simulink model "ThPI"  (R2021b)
settings: Solver=FixedStepAuto  StartTime=0  StopTime=timeWaypoints(end)-0.2  FixedStep=0.005  RelTol=1e-3
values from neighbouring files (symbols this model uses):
  a = 0.27    [CompareGazeboSimulink.m]    (also in RobotModel.m)
  b = 0.31    [CompareGazeboSimulink.m]    (also in RobotModel.m)
  D = abs(a-b)    [RobotModel.m]
  Dflag = 1    [RobotModel.m]
  distAng = 0    [RobotModel.m]
  distVel = 0    [RobotModel.m]
  fro = 0.02    [CompareGazeboSimulink.m]    (also in RobotModel.m)
  fsl = 0.8    [CompareGazeboSimulink.m]    (also in RobotModel.m)
  fsly = 0.8    [CompareGazeboSimulink.m]    (also in RobotModel.m)
  I = (1/12)*m*((2*t)^2 + 0.12^2) + 1.5    (= 2.384)    [CompareGazeboSimulink.m]    (also in RobotModel.m = 0.866666666667)
  Iflag = 1    [RobotModel.m]
  K = 22    [RobotModel.m]
  ko = 0    [CompareGazeboSimulink.m]    (also in RobotModel.m = 0.25)
  kt = 0.58    [CompareGazeboSimulink.m]    (also in RobotModel.m)
  kx = 0.5    [RobotModel.m]
  ky = 0.5    [RobotModel.m]
  lx = 0.15    [RobotModel.m]
  ly = 0.15    [RobotModel.m]
  m = 51    [CompareGazeboSimulink.m]    (also in RobotModel.m = 50)
  mdy = 10    [CompareGazeboSimulink.m]    (also in RobotModel.m)
  mst = 10    [CompareGazeboSimulink.m]    (also in RobotModel.m)
  N = 0    [RobotModel.m]
  r = 0.19    [CompareGazeboSimulink.m]    (also in RobotModel.m)
  T_vel_variance = 0.0005    [RobotModel.m]
  Td = 0.0125    [RobotModel.m]
  Th0 = 0    [CompareGazeboSimulink.m]    (also in RobotModel.m = 0.9714)
  Th_vel0 = 0    [CompareGazeboSimulink.m]    (also in RobotModel.m)
  Ti = 0.1    [RobotModel.m]
  timeWaypoints = [0, 3, 7.5, 10.5, 13.5, 18, 20.5]    [RobotModel.m]
  Ts = 0.01    [CompareGazeboSimulink.m]    (also in RobotModel.m = 0.05)
  waypoints = [0 5; 4 9; 8 1; 12 5; 8 9; 4 1; 0 5]    [CubicSpline.m]    (also in RobotModel.m = [0 2.5; 2 4.5; 4 0.5; 6 2.5; 4 4.5; 2 0.5; 0 2.5])
  X0 = 0    [CompareGazeboSimulink.m]    (also in RobotModel.m)
  x_vel0 = 0    [CompareGazeboSimulink.m]    (also in RobotModel.m)
  x_vel_variance = 0.0005    [RobotModel.m]
  Y0 = 0    [CompareGazeboSimulink.m]    (also in RobotModel.m = 2.5)

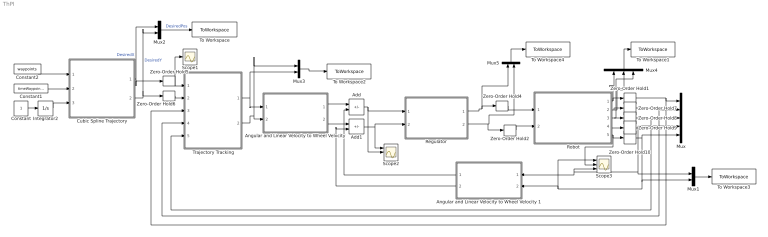
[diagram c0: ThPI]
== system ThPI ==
  Add : Sum  Inputs=+-
  Add1 : Sum  Inputs=+-
  Angular and Linear Velocity to Wheel Velocity : Subsystem
  Angular and Linear Velocity to Wheel Velocity 1 : Subsystem
  Constant : Constant
  Constant1 : Constant  Value=timeWaypoints
  Constant2 : Constant  Value=waypoints
  Cubic Spline Trajectory : MATLAB Function  TreatAsAtomicUnit=on
  Integrator2 : Integrator
  Mux : Mux  Inputs=5
  Mux{1..3,5} (4 alike) : Mux  Inputs=2
  Mux4 : Mux  Inputs=3
  Regulator : Subsystem
  Robot : Subsystem
  Scope1 : Scope
  Scope2 : Scope  NumInputPorts=3
  Scope3 : Scope  NumInputPorts=3
  To Workspace : ToWorkspace  VariableName=desiredPos  SaveFormat=Timeseries  SampleTime=-1
  To Workspace1 : ToWorkspace  VariableName=ActualPos  SaveFormat=Timeseries  SampleTime=-1
  To Workspace2 : ToWorkspace  VariableName=DesiredVel  SaveFormat=Timeseries  SampleTime=-1
  To Workspace3 : ToWorkspace  VariableName=ActualVel  SaveFormat=Timeseries  SampleTime=-1
  To Workspace4 : ToWorkspace  VariableName=Forces  SaveFormat=Timeseries  SampleTime=-1
  Trajectory Tracking : Subsystem
  Zero-Order Hold{1..2,4..10} (9 alike) : ZeroOrderHold  SampleTime=Ts
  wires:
  Angular and Linear Velocity to Wheel Velocity 1/1(wl) -> Add/2
  Angular and Linear Velocity to Wheel Velocity 1/2("wr ") -> Add1/2
  Constant2/1 -> Cubic Spline Trajectory/1(waypoints)
  Constant/1 -> Integrator2/1
  Constant1/1 -> Cubic Spline Trajectory/2(time)
  Integrator2/1 -> Cubic Spline Trajectory/3(actualTime)
  Cubic Spline Trajectory/1(X) -> Mux2/1, Zero-Order Hold5/1  "DesiredX"
  Cubic Spline Trajectory/2(Y) -> Zero-Order Hold6/1, Mux2/2  "DesiredY"
  Add/1 -> Scope2/2, Regulator/1(wl)
  Add1/1 -> Scope2/1, Regulator/2(wr)
  Regulator/2(Right force action) -> Mux5/2, Zero-Order Hold2/1
  Regulator/1(Left Force action) -> Mux5/1, Zero-Order Hold4/1
  Angular and Linear Velocity to Wheel Velocity/1(wl) -> Add/1
  Angular and Linear Velocity to Wheel Velocity/2("wr ") -> Add1/1
  Zero-Order Hold4/1 -> Robot/1(Left Force)
  Zero-Order Hold2/1 -> Robot/2(Right Force)
  Mux2/1 -> To Workspace/1  "DesiredPos"
  Zero-Order Hold5/1 -> Scope1/1, Trajectory Tracking/1(Xd)
  Zero-Order Hold6/1 -> Trajectory Tracking/2(Yd)
  Mux4/1 -> To Workspace1/1
  Robot/1(X) -> Mux4/1, Zero-Order Hold1/1
  Robot/2(Y) -> Mux4/2, Zero-Order Hold7/1
  Robot/5(v) -> Scope3/2, Zero-Order Hold10/1
  Zero-Order Hold8/1 -> Trajectory Tracking/5(Theta), Mux/3
  Zero-Order Hold10/1 -> Scope3/1, Angular and Linear Velocity to Wheel Velocity 1/2(Linear Velocity), Mux1/2, Mux/5
  Zero-Order Hold9/1 -> Scope3/3, Angular and Linear Velocity to Wheel Velocity 1/1(Angular Velocity), Mux1/1, Mux/4
  Zero-Order Hold1/1 -> Trajectory Tracking/3(X), Mux/1
  Zero-Order Hold7/1 -> Trajectory Tracking/4(Y), Mux/2
  Robot/3(Theta) -> Mux4/3, Zero-Order Hold8/1
  Robot/4(Theta') -> Zero-Order Hold9/1
  Mux5/1 -> To Workspace4/1
  Mux1/1 -> To Workspace3/1
  Mux3/1 -> To Workspace2/1
  Trajectory Tracking/1(" Linear Velocity") -> Mux3/2, Angular and Linear Velocity to Wheel Velocity/1(Linear Velocity)
  Trajectory Tracking/2(Angular Velocity) -> Mux3/1, Angular and Linear Velocity to Wheel Velocity/2(Angular Velocity)

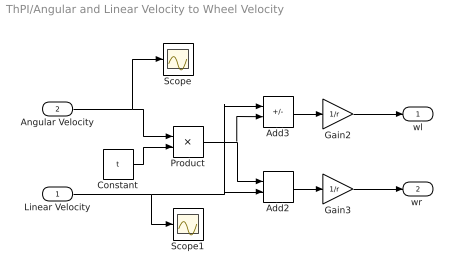
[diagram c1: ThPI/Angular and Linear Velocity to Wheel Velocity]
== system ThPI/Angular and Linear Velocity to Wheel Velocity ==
  Linear Velocity : Inport
  Angular Velocity : Inport  Port=2
  Add2 : Sum
  Add3 : Sum  Inputs=+-
  Constant : Constant  Value=t
  Gain2 : Gain  Gain=1/r
  Gain3 : Gain  Gain=1/r
  Product : Product
  Scope : Scope
  Scope1 : Scope
  wl : Outport
  "wr " : Outport  Port=2
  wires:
  Gain2/1 -> wl/1
  Linear Velocity/1 -> Scope1/1, Add2/2, Add3/1
  Gain3/1 -> "wr "/1
  Product/1 -> Add3/2, Add2/1
  Constant/1 -> Product/2
  Add3/1 -> Gain2/1
  Add2/1 -> Gain3/1
  Angular Velocity/1 -> Scope/1, Product/1

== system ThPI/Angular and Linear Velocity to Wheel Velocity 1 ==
  Angular Velocity : Inport
  Linear Velocity : Inport  Port=2
  Add2 : Sum
  Add3 : Sum  Inputs=+-
  Constant : Constant  Value=t
  Gain2 : Gain  Gain=1/r
  Gain3 : Gain  Gain=1/r
  Product : Product
  wl : Outport
  "wr " : Outport  Port=2
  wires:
  Angular Velocity/1 -> Product/1
  Add2/1 -> Gain3/1
  Add3/1 -> Gain2/1
  Constant/1 -> Product/2
  Product/1 -> Add2/1, Add3/2
  Gain3/1 -> "wr "/1
  Linear Velocity/1 -> Add3/1, Add2/2
  Gain2/1 -> wl/1

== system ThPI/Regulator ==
  wl : Inport
  wr : Inport  Port=2
  PSDN : Subsystem
  PSDN1 : Subsystem
  Left Force action : Outport
  Right force action : Outport  Port=2
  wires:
  wl/1 -> PSDN/1(wl)
  PSDN/1(Left Force action) -> Left Force action/1
  wr/1 -> PSDN1/1(wr)
  PSDN1/1(Right force action) -> Right force action/1

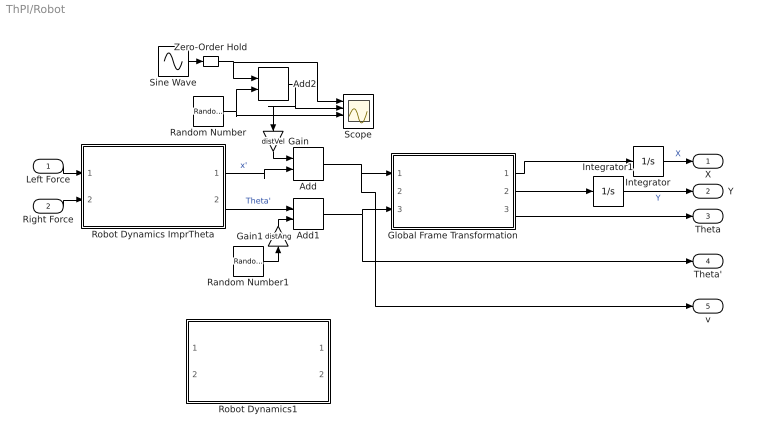
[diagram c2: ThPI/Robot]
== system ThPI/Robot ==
  Left Force : Inport
  Right Force : Inport  Port=2
  Add : Sum
  Add1 : Sum
  Add2 : Sum
  Gain : Gain  Gain=distVel
  Gain1 : Gain  Gain=distAng
  Global Frame Transformation : Subsystem
  Integrator : Integrator  InitialCondition=X0
  Integrator1 : Integrator  InitialCondition=Y0
  Random Number : RandomNumber  Variance=x_vel_variance  SampleTime=0.5
  Random Number1 : RandomNumber  Variance=T_vel_variance  SampleTime=0.1
  Robot Dynamics ImprTheta : Subsystem
  Robot Dynamics1 : Subsystem  Commented=on
  Scope : Scope  NumInputPorts=4
  Sine Wave : Sin  Amplitude=0.1  Frequency=0.2  SampleTime=0
  Zero-Order Hold : ZeroOrderHold  SampleTime=0.25
  X : Outport
  Y : Outport  Port=2
  Theta : Outport  Port=3
  Theta' : Outport  Port=4
  v : Outport  Port=5
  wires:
  Random Number/1 -> Add2/2, Scope/3
  Add2/1 -> Gain/1, Scope/2
  Gain/1 -> Add/1
  Sine Wave/1 -> Zero-Order Hold/1
  Add/1 -> v/1, Global Frame Transformation/1(x')
  Add1/1 -> Theta'/1, Global Frame Transformation/3(Theta')
  Random Number1/1 -> Gain1/1
  Left Force/1 -> Robot Dynamics ImprTheta/1(Left Force)
  Gain1/1 -> Add1/2
  Integrator1/1 -> Y/1  "Y"
  Zero-Order Hold/1 -> Scope/1, Add2/1
  Robot Dynamics ImprTheta/1(x') -> Add/2  "x'"
  Global Frame Transformation/2(Y') -> Integrator1/1
  Integrator/1 -> X/1  "X"
  Right Force/1 -> Robot Dynamics ImprTheta/2(Right Force)
  Global Frame Transformation/1(X') -> Integrator/1
  Global Frame Transformation/3(Theta) -> Theta/1
  Robot Dynamics ImprTheta/2(Theta') -> Add1/1  "Theta'"

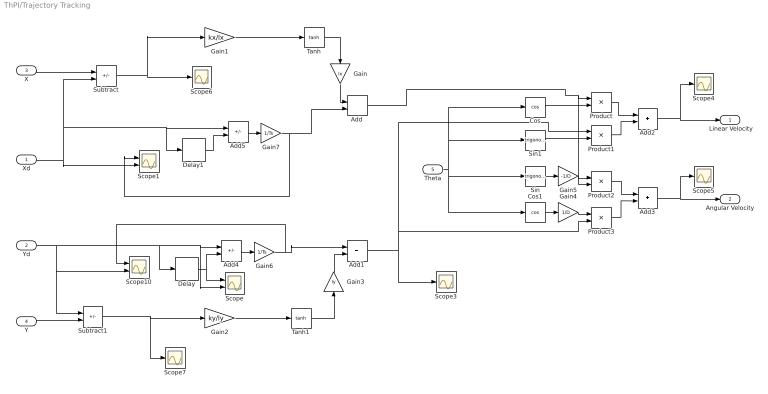
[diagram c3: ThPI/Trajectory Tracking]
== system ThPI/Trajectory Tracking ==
  Xd : Inport
  Yd : Inport  Port=2
  X : Inport  Port=3
  Y : Inport  Port=4
  Theta : Inport  Port=5
  Add{,1..3} (4 alike) : Sum
  Add4 : Sum  Inputs=+-
  Add5 : Sum  Inputs=+-
  Cos : Trigonometry  Operator=cos
  Cos1 : Trigonometry  Operator=cos
  Delay : Delay  DelayLength=1  InitialCondition=Y0
  Delay1 : Delay  DelayLength=1  InitialCondition=X0
  Gain : Gain  Gain=lx
  Gain1 : Gain  Gain=kx/lx
  Gain2 : Gain  Gain=ky/ly
  Gain3 : Gain  Gain=ly
  Gain4 : Gain  Gain=1/D
  Gain5 : Gain  Gain=-1/D
  Gain6 : Gain  Gain=1/Ts
  Gain7 : Gain  Gain=1/Ts
  Product{,1..3} (4 alike) : Product
  Scope : Scope  NumInputPorts=2
  Scope1 : Scope  NumInputPorts=2
  Scope10 : Scope  NumInputPorts=2
  Scope{3..7} (5 alike) : Scope
  Sin : Trigonometry
  Sin1 : Trigonometry
  Subtract : Sum  Inputs=-+
  Subtract1 : Sum  Inputs=+-
  Tanh : Trigonometry  Operator=tanh
  Tanh1 : Trigonometry  Operator=tanh
  " Linear Velocity" : Outport
  Angular Velocity : Outport  Port=2
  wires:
  Subtract/1 -> Gain1/1, Scope6/1
  Subtract1/1 -> Scope7/1, Gain2/1
  Add4/1 -> Gain6/1
  Tanh/1 -> Gain/1
  Gain1/1 -> Tanh/1
  Gain2/1 -> Tanh1/1
  Tanh1/1 -> Gain3/1
  Cos1/1 -> Gain4/1
  Sin/1 -> Gain5/1
  Theta/1 -> Cos/1, Sin1/1, Cos1/1, Sin/1
  Cos/1 -> Product/2
  Add/1 -> Product2/2, Product/1
  Sin1/1 -> Product1/2
  Gain5/1 -> Product2/1
  Gain4/1 -> Product3/1
  Add1/1 -> Scope3/1, Product3/2, Product1/1
  Product/1 -> Add2/1
  Product1/1 -> Add2/2
  Product2/1 -> Add3/1
  Product3/1 -> Add3/2
  Add2/1 -> Scope4/1, " Linear Velocity"/1
  Add3/1 -> Scope5/1, Angular Velocity/1
  Y/1 -> Subtract1/2
  Yd/1 -> Delay/1, Add4/1, Scope/2, Scope10/2, Subtract1/1
  X/1 -> Subtract/1
  Gain/1 -> Add/1
  Gain3/1 -> Add1/2
  Delay/1 -> Scope/1, Add4/2
  Gain6/1 -> Scope10/1, Add1/1
  Gain7/1 -> Scope1/1, Add/2
  Delay1/1 -> Add5/2
  Xd/1 -> Scope1/2, Delay1/1, Add5/1, Subtract/2
  Add5/1 -> Gain7/1

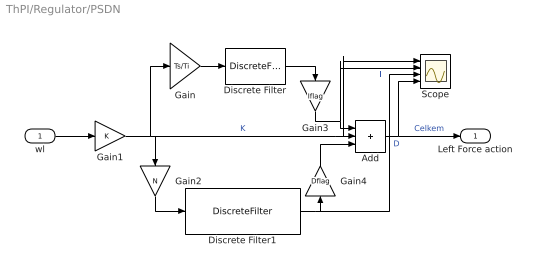
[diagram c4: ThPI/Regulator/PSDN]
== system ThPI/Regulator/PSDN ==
  wl : Inport
  Add : Sum  Inputs=3
  Discrete Filter : DiscreteFilter  Numerator=[0 1]  Denominator=[1 -1]
  Discrete Filter1 : DiscreteFilter  Numerator=[1 -1]  Denominator=[1 -exp(-Ts*N/Td)]
  Gain : Gain  Gain=Ts/Ti
  Gain1 : Gain  Gain=K
  Gain2 : Gain  Gain=N
  Gain3 : Gain  Gain=Iflag
  Gain4 : Gain  Gain=Dflag
  Scope : Scope  NumInputPorts=4
  Left Force action : Outport
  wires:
  Discrete Filter/1 -> Gain3/1
  Discrete Filter1/1 -> Scope/3, Gain4/1  "D"
  wl/1 -> Gain1/1
  Add/1 -> Left Force action/1, Scope/4  "Celkem"
  Gain/1 -> Discrete Filter/1
  Gain1/1 -> Gain2/1, Gain/1, Scope/1, Add/2  "K"
  Gain2/1 -> Discrete Filter1/1
  Gain3/1 -> Scope/2, Add/1  "I"
  Gain4/1 -> Add/3

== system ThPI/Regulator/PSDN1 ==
  wr : Inport
  Add : Sum  Inputs=3
  Discrete Filter : DiscreteFilter  Numerator=[0 1]  Denominator=[1 -1]
  Discrete Filter1 : DiscreteFilter  Numerator=[1 -1]  Denominator=[1 -exp(-Ts*N/Td)]
  Gain : Gain  Gain=Ts/Ti
  Gain1 : Gain  Gain=K
  Gain2 : Gain  Gain=N
  Gain3 : Gain  Gain=Iflag
  Gain4 : Gain  Gain=Dflag
  Right force action : Outport
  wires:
  Gain2/1 -> Discrete Filter1/1
  Gain1/1 -> Add/2, Gain/1, Gain2/1
  Gain/1 -> Discrete Filter/1
  Add/1 -> Right force action/1
  wr/1 -> Gain1/1
  Discrete Filter1/1 -> Gain4/1
  Discrete Filter/1 -> Gain3/1
  Gain3/1 -> Add/1
  Gain4/1 -> Add/3

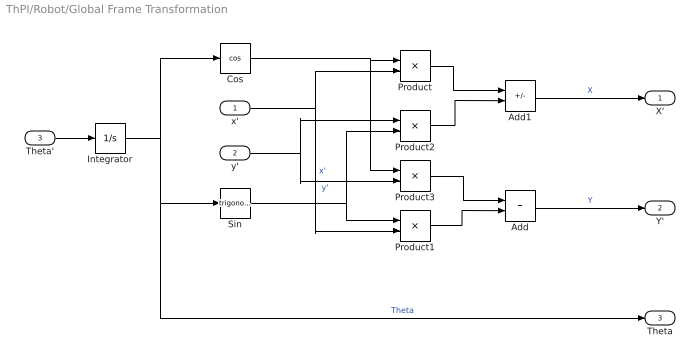
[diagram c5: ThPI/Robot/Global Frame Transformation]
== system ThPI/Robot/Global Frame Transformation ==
  x' : Inport
  y' : Inport  Port=2
  Theta' : Inport  Port=3
  Add : Sum
  Add1 : Sum  Inputs=+-
  Cos : Trigonometry  Operator=cos
  Integrator : Integrator  InitialCondition=Th0
  Product{,1..3} (4 alike) : Product
  Sin : Trigonometry
  X' : Outport
  Y' : Outport  Port=2
  Theta : Outport  Port=3
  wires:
  Add/1 -> Y'/1  "Y"
  Integrator/1 -> Theta/1, Sin/1, Cos/1  "Theta"
  Product1/1 -> Add/2
  x'/1 -> Product/2, Product1/2  "x'"
  Sin/1 -> Product1/1, Product2/2
  Product2/1 -> Add1/2
  Product3/1 -> Add/1
  Product/1 -> Add1/1
  Cos/1 -> Product/1, Product3/1
  y'/1 -> Product3/2, Product2/1  "y'"
  Add1/1 -> X'/1  "X"
  Theta'/1 -> Integrator/1

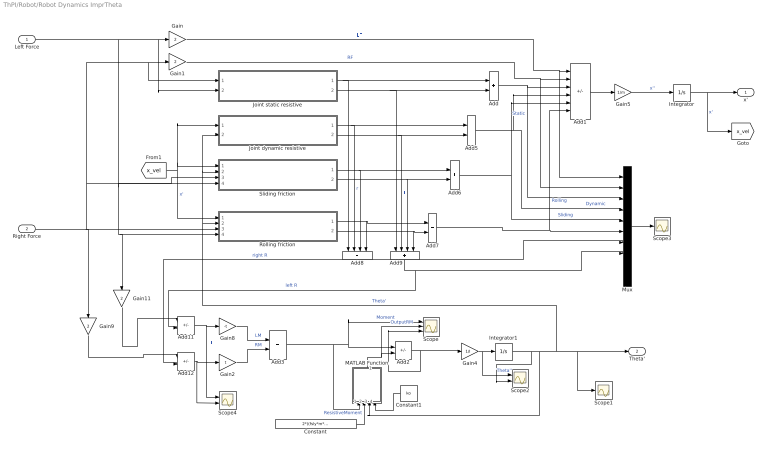
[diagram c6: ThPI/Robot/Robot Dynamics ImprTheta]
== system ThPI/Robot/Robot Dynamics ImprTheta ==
  Left Force : Inport
  Right Force : Inport  Port=2
  Add{,3,5..7} (5 alike) : Sum
  Add1 : Sum  Inputs=++----
  Add11 : Sum  Inputs=+-
  Add12 : Sum  Inputs=+-
  Add2 : Sum  Inputs=+-
  Add8 : Sum  Inputs=++++
  Add9 : Sum  Inputs=++++
  Constant : Constant  Value=2*((fsly*m*9.81)/(a+b))*a*b*kt
  Constant1 : Constant  Value=ko
  Gain{,1,9,11} (4 alike) : Gain  Gain=2
  Gain2 : Gain  Gain=t
  Gain4 : Gain  Gain=1/I
  Gain5 : Gain  Gain=1/m
  Gain8 : Gain  Gain=-t
  Integrator : Integrator  InitialCondition=x_vel0
  Integrator1 : Integrator  InitialCondition=Th_vel0
  Joint dynamic resistive : Subsystem
  Joint static resistive : Subsystem
  MATLAB Function : MATLAB Function  TreatAsAtomicUnit=on
  Mux : Mux  Inputs=10
  Rolling friction : Subsystem
  Scope : Scope  NumInputPorts=3
  Scope1 : Scope
  Scope2 : Scope  NumInputPorts=2
  Scope3 : Scope
  Scope4 : Scope  NumInputPorts=2
  Sliding friction : Subsystem
  x' : Outport
  Theta' : Outport  Port=2
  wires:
  Gain4/1 -> Scope2/1, Integrator1/1  "Theta''"
  Integrator1/1 -> Scope2/2, Sliding friction/2(Theta'), Joint dynamic resistive/2(Theta'), Rolling friction/2(Theta'), Scope1/1, Theta'/1, MATLAB Function/3(Omega)  "Theta'"
  Gain1/1 -> Mux/2, Add1/2  "RF"
  Add1/1 -> Gain5/1
  Gain5/1 -> Integrator/1  "x''"
  Integrator/1 -> x'/1, [x_vel]  "x'"
  [x_vel] -> Joint dynamic resistive/1("Local Long Velocity "), Sliding friction/1(Local longitudal velocity), Rolling friction/1(Local longitudal velocity)  "x'"
  Joint static resistive/2(Static Resistive Force Left) -> Add9/1, Add/2
  Joint dynamic resistive/1(Dynamic Resistive Force Right) -> Add8/2, Add5/1  "r"
  Joint dynamic resistive/2(Dynamic Resistive Force Left) -> Add9/2, Add5/2  "l"
  Sliding friction/1(Friction Right Force) -> Add8/3, Add6/1
  Sliding friction/2(Friction Left Force) -> Add9/3, Add6/2
  Rolling friction/1(Friction Right Force) -> Add8/4, Add7/1
  Rolling friction/2(Friction Left Force) -> Add9/4, Add7/2
  Add/1 -> Add1/3, Mux/3  "Static"
  Add6/1 -> Add1/5, Mux/5  "Sliding"
  Add7/1 -> Mux/6, Add1/6  "Rolling"
  Add5/1 -> Mux/4, Add1/4  "Dynamic"
  Add9/1 -> Add11/2, Mux/8  "left R"
  Add8/1 -> Add12/2, Mux/7  "right R"
  Mux/1 -> Scope3/1
  Add11/1 -> Scope4/1, Gain8/1  "LL"
  Add12/1 -> Scope4/2, Gain2/1
  Gain9/1 -> Add12/1
  Gain11/1 -> Add11/1
  Gain8/1 -> Add3/1  "LM"
  Gain2/1 -> Add3/2  "RM"
  Gain/1 -> Mux/1, Add1/1  "LF"
  Joint static resistive/1(Static Resistive Force Right) -> Add8/1, Add/1
  Add2/1 -> Scope/3, Gain4/1
  Add3/1 -> Scope/1, Add2/1, MATLAB Function/1(Moment)  "Moment"
  MATLAB Function/1(y) -> Scope/2, Add2/2  "OutputRM"
  Constant/1 -> MATLAB Function/2(ResistiveMoment)  "ResistiveMoment"
  Left Force/1 -> Gain11/1, Rolling friction/4(Fl), Sliding friction/4(Fl), Joint static resistive/2("Fl "), Gain/1
  Right Force/1 -> Gain9/1, Rolling friction/3(Fr), Sliding friction/3(Fr), Joint static resistive/1(Fr), Gain1/1
  Constant1/1 -> MATLAB Function/4(ko)

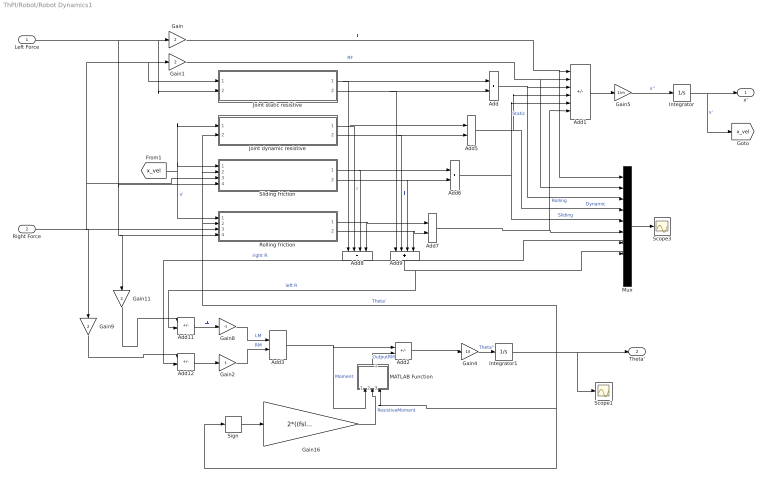
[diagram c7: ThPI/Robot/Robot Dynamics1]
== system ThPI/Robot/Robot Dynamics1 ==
  Left Force : Inport
  Right Force : Inport  Port=2
  Add{,3,5..7} (5 alike) : Sum
  Add1 : Sum  Inputs=++----
  Add11 : Sum  Inputs=+-
  Add12 : Sum  Inputs=+-
  Add2 : Sum  Inputs=+-
  Add8 : Sum  Inputs=++++
  Add9 : Sum  Inputs=++++
  Gain{,1,9,11} (4 alike) : Gain  Gain=2
  Gain16 : Gain  Gain=2*((fsly*m*9.81)/(a+b))*a*b
  Gain2 : Gain  Gain=t
  Gain4 : Gain  Gain=1/I
  Gain5 : Gain  Gain=1/m
  Gain8 : Gain  Gain=-t
  Integrator : Integrator  InitialCondition=x_vel0
  Integrator1 : Integrator  InitialCondition=Th_vel0
  Joint dynamic resistive : Subsystem
  Joint static resistive : Subsystem
  MATLAB Function : MATLAB Function  TreatAsAtomicUnit=on
  Mux : Mux  Inputs=10
  Rolling friction : Subsystem
  Scope1 : Scope
  Scope3 : Scope
  Sign : Signum
  Sliding friction : Subsystem
  x' : Outport
  Theta' : Outport  Port=2
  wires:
  Right Force/1 -> Rolling friction/3(Fr), Sliding friction/3(Fr), Joint static resistive/1(Fr), Gain1/1, Gain9/1
  Gain4/1 -> Integrator1/1  "Theta''"
  Integrator1/1 -> Sliding friction/2(Theta'), Joint dynamic resistive/2(Theta'), Rolling friction/2(Theta'), MATLAB Function/3(Omega), Sign/1, Scope1/1, Theta'/1  "Theta'"
  Left Force/1 -> Rolling friction/4(Fl), Gain11/1, Sliding friction/4(Fl), Joint static resistive/2("Fl "), Gain/1
  Gain1/1 -> Mux/2, Add1/2  "RF"
  Add1/1 -> Gain5/1
  Gain5/1 -> Integrator/1  "x''"
  Integrator/1 -> x'/1, [x_vel]  "x'"
  [x_vel] -> Joint dynamic resistive/1("Local Long Velocity "), Sliding friction/1(Local longitudal velocity), Rolling friction/1(Local longitudal velocity)  "x'"
  Joint static resistive/2(Static Resistive Force Left) -> Add9/1, Add/2
  Joint dynamic resistive/1(Dynamic Resistive Force Right) -> Add8/2, Add5/1  "r"
  Joint dynamic resistive/2(Dynamic Resistive Force Left) -> Add9/2, Add5/2  "l"
  Sliding friction/1(Friction Right Force) -> Add8/3, Add6/1
  Sliding friction/2(Friction Left Force) -> Add9/3, Add6/2
  Rolling friction/1(Friction Right Force) -> Add8/4, Add7/1
  Rolling friction/2(Friction Left Force) -> Add9/4, Add7/2
  Add/1 -> Add1/3, Mux/3  "Static"
  Add6/1 -> Add1/5, Mux/5  "Sliding"
  Add7/1 -> Mux/6, Add1/6  "Rolling"
  Add5/1 -> Mux/4, Add1/4  "Dynamic"
  Add9/1 -> Add11/2, Mux/8  "left R"
  Add8/1 -> Add12/2, Mux/7  "right R"
  Mux/1 -> Scope3/1
  Add11/1 -> Gain8/1  "LL"
  Add12/1 -> Gain2/1
  Gain9/1 -> Add12/1
  Gain11/1 -> Add11/1
  Gain8/1 -> Add3/1  "LM"
  Gain2/1 -> Add3/2  "RM"
  Gain/1 -> Mux/1, Add1/1  "LF"
  Joint static resistive/1(Static Resistive Force Right) -> Add8/1, Add/1
  Sign/1 -> Gain16/1
  Add2/1 -> Gain4/1
  Add3/1 -> Add2/1, MATLAB Function/1(Moment)  "Moment"
  MATLAB Function/1(y) -> Add2/2  "OutputRM"
  Gain16/1 -> MATLAB Function/2(ResistiveMoment)  "ResistiveMoment"

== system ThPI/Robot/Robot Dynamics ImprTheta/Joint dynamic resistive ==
  "Local Long Velocity " : Inport
  Theta' : Inport  Port=2
  Add2 : Sum  Inputs=+-
  Add5 : Sum
  Gain : Gain  Gain=(2*mdy)/(r*r)
  Gain1 : Gain  Gain=(2*mdy)/(r*r)
  Gain4 : Gain  Gain=t
  Scope : Scope  NumInputPorts=3
  Dynamic Resistive Force Right : Outport
  Dynamic Resistive Force Left : Outport  Port=2
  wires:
  Gain/1 -> Dynamic Resistive Force Right/1
  Gain1/1 -> Dynamic Resistive Force Left/1
  Gain4/1 -> Add5/2, Add2/2
  Theta'/1 -> Scope/3, Gain4/1
  Add5/1 -> Scope/2, Gain/1  "vr"
  Add2/1 -> Scope/1, Gain1/1  "vl"
  "Local Long Velocity "/1 -> Add2/1, Add5/1

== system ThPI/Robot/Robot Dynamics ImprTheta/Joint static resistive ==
  Fr : Inport
  "Fl " : Inport  Port=2
  Fsj : Gain  Gain=2*(mst/r)
  Fsj . : Gain  Gain=2*(mst/r)
  Gain1 : Gain  Gain=1/(mst/r)
  Gain2 : Gain  Gain=1/(mst/r)
  Tanh : Trigonometry  Operator=tanh
  Tanh1 : Trigonometry  Operator=tanh
  Static Resistive Force Right : Outport
  Static Resistive Force Left : Outport  Port=2
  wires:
  Fr/1 -> Gain1/1
  "Fl "/1 -> Gain2/1
  Tanh/1 -> Fsj/1
  Tanh1/1 -> Fsj ./1
  Gain1/1 -> Tanh/1
  Gain2/1 -> Tanh1/1
  Fsj/1 -> Static Resistive Force Right/1
  Fsj ./1 -> Static Resistive Force Left/1

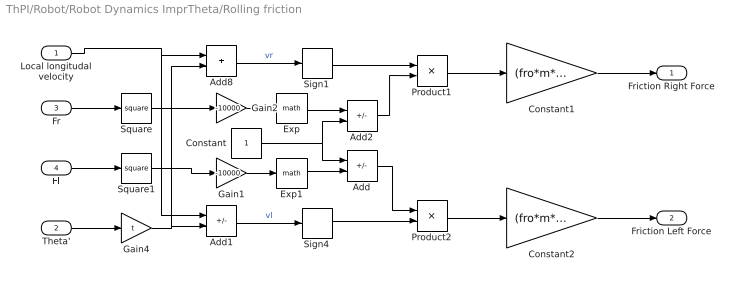
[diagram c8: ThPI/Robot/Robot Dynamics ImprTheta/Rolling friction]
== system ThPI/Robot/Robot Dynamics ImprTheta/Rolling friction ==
  Local longitudal velocity : Inport
  Theta' : Inport  Port=2
  Fr : Inport  Port=3
  Fl : Inport  Port=4
  Add : Sum  Inputs=+-
  Add1 : Sum  Inputs=+-
  Add2 : Sum  Inputs=-+
  Add8 : Sum
  Constant : Constant
  Constant1 : Gain  Gain=(fro*m*9.81)/2
  Constant2 : Gain  Gain=(fro*m*9.81)/2
  Exp : Math
  Exp1 : Math
  Gain1 : Gain  Gain=-10000
  Gain2 : Gain  Gain=-10000
  Gain4 : Gain  Gain=t
  Product1 : Product
  Product2 : Product
  Sign1 : Signum
  Sign4 : Signum
  Square : Math  Operator=square
  Square1 : Math  Operator=square
  Friction Right Force : Outport
  Friction Left Force : Outport  Port=2
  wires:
  Sign1/1 -> Product1/1
  Sign4/1 -> Product2/2
  Add8/1 -> Sign1/1  "vr"
  Fl/1 -> Square1/1
  Fr/1 -> Square/1
  Square1/1 -> Gain1/1
  Gain4/1 -> Add1/2, Add8/2
  Theta'/1 -> Gain4/1
  Add1/1 -> Sign4/1  "vl"
  Square/1 -> Gain2/1
  Gain2/1 -> Exp/1
  Gain1/1 -> Exp1/1
  Add2/1 -> Product1/2
  Add/1 -> Product2/1
  Exp1/1 -> Add/2
  Exp/1 -> Add2/1
  Constant/1 -> Add2/2, Add/1
  Local longitudal velocity/1 -> Add1/1, Add8/1
  Product1/1 -> Constant1/1
  Product2/1 -> Constant2/1
  Constant2/1 -> Friction Left Force/1
  Constant1/1 -> Friction Right Force/1

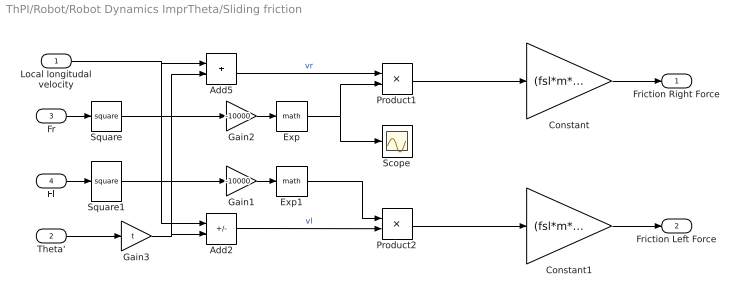
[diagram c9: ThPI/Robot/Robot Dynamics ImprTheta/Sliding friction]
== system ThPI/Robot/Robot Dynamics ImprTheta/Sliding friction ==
  Local longitudal velocity : Inport
  Theta' : Inport  Port=2
  Fr : Inport  Port=3
  Fl : Inport  Port=4
  Add2 : Sum  Inputs=+-
  Add5 : Sum
  Constant : Gain  Gain=(fsl*m*9.81)/2
  Constant1 : Gain  Gain=(fsl*m*9.81)/2
  Exp : Math
  Exp1 : Math
  Gain1 : Gain  Gain=-10000
  Gain2 : Gain  Gain=-10000
  Gain3 : Gain  Gain=t
  Product1 : Product
  Product2 : Product
  Scope : Scope
  Square : Math  Operator=square
  Square1 : Math  Operator=square
  Friction Right Force : Outport
  Friction Left Force : Outport  Port=2
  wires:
  Theta'/1 -> Gain3/1
  Gain3/1 -> Add2/2, Add5/2
  Add5/1 -> Product1/1  "vr"
  Add2/1 -> Product2/2  "vl"
  Exp/1 -> Scope/1, Product1/2
  Gain1/1 -> Exp1/1
  Gain2/1 -> Exp/1
  Fr/1 -> Square/1
  Fl/1 -> Square1/1
  Square/1 -> Gain2/1
  Square1/1 -> Gain1/1
  Product1/1 -> Constant/1
  Product2/1 -> Constant1/1
  Exp1/1 -> Product2/1
  Local longitudal velocity/1 -> Add2/1, Add5/1
  Constant/1 -> Friction Right Force/1
  Constant1/1 -> Friction Left Force/1

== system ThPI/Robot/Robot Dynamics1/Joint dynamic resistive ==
  "Local Long Velocity " : Inport
  Theta' : Inport  Port=2
  Add2 : Sum  Inputs=+-
  Add5 : Sum
  Gain : Gain  Gain=(2*mdy)/(r*r)
  Gain1 : Gain  Gain=(2*mdy)/(r*r)
  Gain4 : Gain  Gain=t
  Scope : Scope  NumInputPorts=3
  Dynamic Resistive Force Right : Outport
  Dynamic Resistive Force Left : Outport  Port=2
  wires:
  Gain/1 -> Dynamic Resistive Force Right/1
  Gain1/1 -> Dynamic Resistive Force Left/1
  Gain4/1 -> Add5/2, Add2/2
  Theta'/1 -> Scope/3, Gain4/1
  Add5/1 -> Scope/2, Gain/1  "vr"
  Add2/1 -> Scope/1, Gain1/1  "vl"
  "Local Long Velocity "/1 -> Add2/1, Add5/1

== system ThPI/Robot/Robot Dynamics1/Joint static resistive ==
  Fr : Inport
  "Fl " : Inport  Port=2
  Fsj : Gain  Gain=2*(mst/r)
  Fsj . : Gain  Gain=2*(mst/r)
  Gain1 : Gain  Gain=1/(mst/r)
  Gain2 : Gain  Gain=1/(mst/r)
  Tanh : Trigonometry  Operator=tanh
  Tanh1 : Trigonometry  Operator=tanh
  Static Resistive Force Right : Outport
  Static Resistive Force Left : Outport  Port=2
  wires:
  Fr/1 -> Gain1/1
  "Fl "/1 -> Gain2/1
  Tanh/1 -> Fsj/1
  Tanh1/1 -> Fsj ./1
  Gain1/1 -> Tanh/1
  Gain2/1 -> Tanh1/1
  Fsj/1 -> Static Resistive Force Right/1
  Fsj ./1 -> Static Resistive Force Left/1

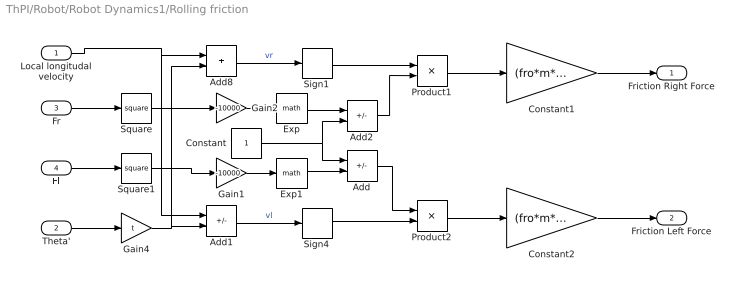
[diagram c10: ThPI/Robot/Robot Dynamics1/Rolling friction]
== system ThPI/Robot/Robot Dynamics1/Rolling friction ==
  Local longitudal velocity : Inport
  Theta' : Inport  Port=2
  Fr : Inport  Port=3
  Fl : Inport  Port=4
  Add : Sum  Inputs=+-
  Add1 : Sum  Inputs=+-
  Add2 : Sum  Inputs=-+
  Add8 : Sum
  Constant : Constant
  Constant1 : Gain  Gain=(fro*m*9.81)/2
  Constant2 : Gain  Gain=(fro*m*9.81)/2
  Exp : Math
  Exp1 : Math
  Gain1 : Gain  Gain=-10000
  Gain2 : Gain  Gain=-10000
  Gain4 : Gain  Gain=t
  Product1 : Product
  Product2 : Product
  Sign1 : Signum
  Sign4 : Signum
  Square : Math  Operator=square
  Square1 : Math  Operator=square
  Friction Right Force : Outport
  Friction Left Force : Outport  Port=2
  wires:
  Sign1/1 -> Product1/1
  Sign4/1 -> Product2/2
  Add8/1 -> Sign1/1  "vr"
  Fl/1 -> Square1/1
  Fr/1 -> Square/1
  Square1/1 -> Gain1/1
  Gain4/1 -> Add1/2, Add8/2
  Theta'/1 -> Gain4/1
  Add1/1 -> Sign4/1  "vl"
  Square/1 -> Gain2/1
  Gain2/1 -> Exp/1
  Gain1/1 -> Exp1/1
  Add2/1 -> Product1/2
  Add/1 -> Product2/1
  Exp1/1 -> Add/2
  Exp/1 -> Add2/1
  Constant/1 -> Add2/2, Add/1
  Local longitudal velocity/1 -> Add1/1, Add8/1
  Product1/1 -> Constant1/1
  Product2/1 -> Constant2/1
  Constant2/1 -> Friction Left Force/1
  Constant1/1 -> Friction Right Force/1

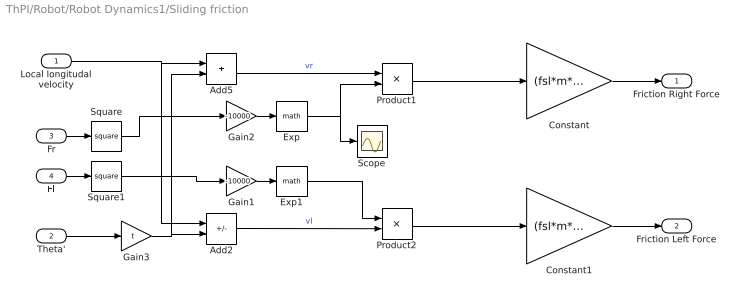
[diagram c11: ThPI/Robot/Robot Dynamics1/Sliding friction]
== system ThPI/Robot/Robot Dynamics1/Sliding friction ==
  Local longitudal velocity : Inport
  Theta' : Inport  Port=2
  Fr : Inport  Port=3
  Fl : Inport  Port=4
  Add2 : Sum  Inputs=+-
  Add5 : Sum
  Constant : Gain  Gain=(fsl*m*9.81)/2
  Constant1 : Gain  Gain=(fsl*m*9.81)/2
  Exp : Math
  Exp1 : Math
  Gain1 : Gain  Gain=-10000
  Gain2 : Gain  Gain=-10000
  Gain3 : Gain  Gain=t
  Product1 : Product
  Product2 : Product
  Scope : Scope
  Square : Math  Operator=square
  Square1 : Math  Operator=square
  Friction Right Force : Outport
  Friction Left Force : Outport  Port=2
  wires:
  Theta'/1 -> Gain3/1
  Gain3/1 -> Add2/2, Add5/2
  Add5/1 -> Product1/1  "vr"
  Add2/1 -> Product2/2  "vl"
  Exp/1 -> Scope/1, Product1/2
  Gain1/1 -> Exp1/1
  Gain2/1 -> Exp/1
  Fr/1 -> Square/1
  Fl/1 -> Square1/1
  Square/1 -> Gain2/1
  Square1/1 -> Gain1/1
  Product1/1 -> Constant/1
  Product2/1 -> Constant1/1
  Exp1/1 -> Product2/1
  Local longitudal velocity/1 -> Add2/1, Add5/1
  Constant/1 -> Friction Right Force/1
  Constant1/1 -> Friction Left Force/1

== matlab function ThPI/Cubic Spline
Trajectory ==
function [X, Y] = TrajectoryGeneration(waypoints, time, actualTime)
%% Cubic spline
t = time;
Ax = zeros((size(waypoints,1)-1)*4);
Bx = zeros((size(waypoints,1)-1)*4, 1);

Ay = zeros((size(waypoints,1)-1)*4);
By = zeros((size(waypoints,1)-1)*4, 1);

%% Start and End Points (1-10)
% First polynom
Ax(1,1:4) = [t(1)^3 t(1)^2 t(1) 1];
Ax(2,1:4) = [t(2)^3 t(2)^2 t(2) 1];
Bx(1) = waypoints(1,1);
Bx(2) = waypoints(2,1);

Ay(1,1:4) = [t(1)^3 t(1)^2 t(1) 1];
Ay(2,1:4) = [t(2)^3 t(2)^2 t(2) 1];
By(1) = waypoints(1,2);
By(2) = waypoints(2,2);

% Second polynom
Ax(3,5:8) = [t(2)^3 t(2)^2 t(2) 1];
Ax(4,5:8) = [t(3)^3 t(3)^2 t(3) 1];
Bx(3) = waypoints(2,1);
Bx(4) = waypoints(3,1);

Ay(3,5:8) = [t(2)^3 t(2)^2 t(2) 1];
Ay(4,5:8) = [t(3)^3 t(3)^2 t(3) 1];
By(3) = waypoints(2,2);
By(4) = waypoints(3,2);

% Third polynom
Ax(5,9:12) = [t(3)^3 t(3)^2 t(3) 1];
Ax(6,9:12) = [t(4)^3 t(4)^2 t(4) 1];
Bx(5) = waypoints(3,1);
Bx(6) = waypoints(4,1);

Ay(5,9:12) = [t(3)^3 t(3)^2 t(3) 1];
Ay(6,9:12) = [t(4)^3 t(4)^2 t(4) 1];
By(5) = waypoints(3,2);
By(6) = waypoints(4,2);

% Fourth polynom
Ax(7,13:16) = [t(4)^3 t(4)^2 t(4) 1];
Ax(8,13:16) = [t(5)^3 t(5)^2 t(5) 1];
Bx(7) = waypoints(4,1);
Bx(8) = waypoints(5,1);

Ay(7,13:16) = [t(4)^3 t(4)^2 t(4) 1];
Ay(8,13:16) = [t(5)^3 t(5)^2 t(5) 1];
By(7) = waypoints(4,2);
By(8) = waypoints(5,2);

% Fifth polynom
Ax(9,17:20) = [t(5)^3 t(5)^2 t(5) 1];
Ax(10,17:20) = [t(6)^3 t(6)^2 t(6) 1];
Bx(9) = waypoints(5,1);
Bx(10) = waypoints(6,1);

Ay(9,17:20) = [t(5)^3 t(5)^2 t(5) 1];
Ay(10,17:20) = [t(6)^3 t(6)^2 t(6) 1];
By(9) = waypoints(5,2);
By(10) = waypoints(6,2);

% Sixth polynom
Ax(11,21:24) = [t(6)^3 t(6)^2 t(6) 1];
Ax(12,21:24) = [t(7)^3 t(7)^2 t(7) 1];
Bx(11) = waypoints(6,1);
Bx(12) = waypoints(7,1);

Ay(11,21:24) = [t(6)^3 t(6)^2 t(6) 1];
Ay(12,21:24) = [t(7)^3 t(7)^2 t(7) 1];
By(11) = waypoints(6,2);
By(12) = waypoints(7,2);

%% First derivation (11-14)
Ax(13, 1:8) = [3*t(2)^2 2*t(2) 1 0 -3*t(2)^2 -2*t(2) -1 0];
Ax(14, 5:12) = [3*t(3)^2 2*t(3) 1 0 -3*t(3)^2 -2*t(3) -1 0];
Ax(15, 9:16) = [3*t(4)^2 2*t(4) 1 0 -3*t(4)^2 -2*t(4) -1 0];
Ax(16, 13:20) = [3*t(5)^2 2*t(5) 1 0 -3*t(5)^2 -2*t(5) -1 0];
Ax(17, 17:24) = [3*t(6)^2 2*t(6) 1 0 -3*t(6)^2 -2*t(6) -1 0];

Ay(13, 1:8) = [3*t(2)^2 2*t(2) 1 0 -3*t(2)^2 -2*t(2) -1 0];
Ay(14, 5:12) = [3*t(3)^2 2*t(3) 1 0 -3*t(3)^2 -2*t(3) -1 0];
Ay(15, 9:16) = [3*t(4)^2 2*t(4) 1 0 -3*t(4)^2 -2*t(4) -1 0];
Ay(16, 13:20) = [3*t(5)^2 2*t(5) 1 0 -3*t(5)^2 -2*t(5) -1 0];
Ay(17, 17:24) = [3*t(6)^2 2*t(6) 1 0 -3*t(6)^2 -2*t(6) -1 0];

%% Second derivation (15-18)
Ax(18, 1:8) = [6*t(2) 2 0 0 -6*t(2) -2 0 0];
Ax(19, 5:12) = [6*t(3) 2 0 0 -6*t(3) -2 0 0];
Ax(20, 9:16) = [6*t(4) 2 0 0 -6*t(4) -2 0 0];
Ax(21, 13:20) = [6*t(5) 2 0 0 -6*t(5) -2 0 0];
Ax(22, 17:24) = [6*t(6) 2 0 0 -6*t(6) -2 0 0];

Ay(18, 1:8) = [6*t(2) 2 0 0 -6*t(2) -2 0 0];
Ay(19, 5:12) = [6*t(3) 2 0 0 -6*t(3) -2 0 0];
Ay(20, 9:16) = [6*t(4) 2 0 0 -6*t(4) -2 0 0];
Ay(21, 13:20) = [6*t(5) 2 0 0 -6*t(5) -2 0 0];
Ay(22, 17:24) = [6*t(6) 2 0 0 -6*t(6) -2 0 0];

%% Initial condition (19-20)
Ax(23, 1:4) = [3*t(1)^2 2*t(1) 1 0];
Ax(24, 21:24) = [3*t(end)^2 2*t(end) 1 0];
Bx(23) = 0;
Bx(24) = 0;

Ay(23, 1:4) = [3*t(1)^2 2*t(1) 1 0];
Ay(24, 21:24) = [3*t(end)^2 2*t(end) 1 0];
By(23) = 0;
By(24) = 0;

%% Solve equation
Px = Ax \ Bx;
Py = Ay \ By;

if(actualTime <= t(2))
    X = [actualTime^3 actualTime^2 actualTime 1]*Px(1:4);
    Y = [actualTime^3 actualTime^2 actualTime 1]*Py(1:4);
elseif(actualTime <= t(3))
    X = [actualTime^3 actualTime^2 actualTime 1]*Px(5:8);
    Y = [actualTime^3 actualTime^2 actualTime 1]*Py(5:8);
elseif(actualTime <= t(4))
    X = [actualTime^3 actualTime^2 actualTime 1]*Px(9:12);
    Y = [actualTime^3 actualTime^2 actualTime 1]*Py(9:12);
elseif(actualTime <= t(5))
    X = [actualTime^3 actualTime^2 actualTime 1]*Px(13:16);
    Y = [actualTime^3 actualTime^2 actualTime 1]*Py(13:16);
elseif(actualTime <= t(6))
    X = [actualTime^3 actualTime^2 actualTime 1]*Px(17:20);
    Y = [actualTime^3 actualTime^2 actualTime 1]*Py(17:20);
else
    X = [actualTime^3 actualTime^2 actualTime 1]*Px(21:24);
    Y = [actualTime^3 actualTime^2 actualTime 1]*Py(21:24);
end     


end

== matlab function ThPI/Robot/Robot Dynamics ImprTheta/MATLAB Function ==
function y = fcn(Moment, ResistiveMoment, Omega, ko)
    y = Omega*ResistiveMoment;

%     if(abs(Moment) < abs(ResistiveMoment))
%         y = Moment;
%     else
%         y = (ko*Omega + sign(Omega))*ResistiveMoment;
%     end



end

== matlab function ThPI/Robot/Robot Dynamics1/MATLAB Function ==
function y = fcn(Moment, ResistiveMoment, Omega)
    y = ResistiveMoment;
    
    if(Omega ~= 0)
        if(abs(Moment) < abs(ResistiveMoment))
            y = sign(Omega)*abs(Moment);
        else
            y = ResistiveMoment;
        end
    else
        y = 0;


end
